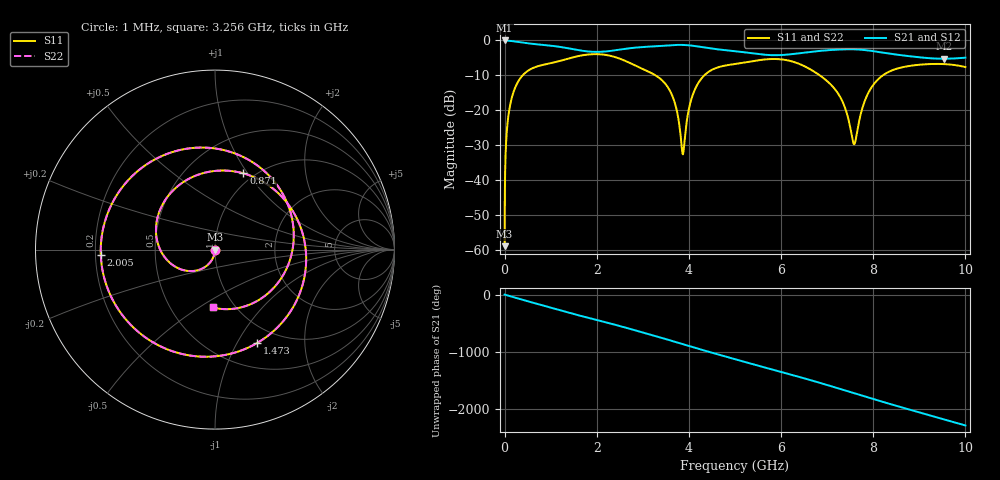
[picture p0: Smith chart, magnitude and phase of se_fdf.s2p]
!Created with skrf (http://scikit-rf.org).
# GHz S RI R 50.0
!freq ReS11 ImS11 ReS21 ImS21 ReS12 ImS12 ReS22 ImS22
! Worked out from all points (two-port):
!   10000 points, 1 MHz to 10 GHz, reference 50 ohm
!   highest |S21| = 0.00 dB at 1 MHz (marker M1); lowest = -5.2 dB at 9.53 GHz (marker M2)
!   |S21| within 3 dB of the highest: start of sweep to 1.716 GHz; 2.294 GHz to 4.951 GHz (2.657 GHz wide, 73.3 % of centre)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
!   lowest |S11| = -58.8 dB at 1 MHz (marker M3), VSWR 1.00, Z = 50 - j0.114 ohm
!   |S11| at or under -10 dB: start of sweep to 391.1 MHz; 3.278 GHz to 4.333 GHz (1.055 GHz wide, 27.7 % of centre); 6.842 GHz to 8.207 GHz (1.366 GHz wide, 18.1 % of centre)
!   |S22| runs from -58.8 to -3.9 dB; largest |S21 - S12| = 1.1e-15
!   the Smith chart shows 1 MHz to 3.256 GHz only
!   S11 on the Smith chart (normalised r, x): 1 MHz: 1.00, -0.00; 871 MHz: 0.89, +0.96; 1.473 GHz: 0.79, -1.22; 2.005 GHz: 0.22, -0.02; 3.256 GHz: 0.79, -0.57
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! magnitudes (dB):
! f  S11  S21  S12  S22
! 1 MHz  -58.8  0.0  0.0  -58.8
! 65 MHz  -23.6  -0.1  -0.1  -23.6
! 176 MHz  -15.5  -0.2  -0.2  -15.5
! 427 MHz  -9.5  -0.7  -0.7  -9.5
! 871 MHz  -6.9  -1.3  -1.3  -6.9
! 1.473 GHz  -4.9  -2.5  -2.5  -4.9
! 1.668 GHz  -4.3  -2.9  -2.9  -4.3
! 2.005 GHz  -3.9  -3.3  -3.3  -3.9
! 3.256 GHz  -9.8  -1.7  -1.7  -9.8
! 3.334 GHz  -10.5  -1.6  -1.6  -10.5
! 3.662 GHz  -16.6  -1.3  -1.3  -16.6
! 3.869 GHz  -32.6  -1.3  -1.3  -32.6
! 4.029 GHz  -18.0  -1.4  -1.4  -18.0
! 4.216 GHz  -11.9  -1.8  -1.8  -11.9
! 5.001 GHz  -6.7  -3.1  -3.1  -6.7
! 6.667 GHz  -8.5  -3.2  -3.2  -8.5
! 7.262 GHz  -15.7  -2.6  -2.6  -15.7
! 7.585 GHz  -29.7  -2.5  -2.5  -29.7
! 7.888 GHz  -15.1  -2.9  -2.9  -15.1
! 8.334 GHz  -9.0  -3.7  -3.7  -9.0
! 9.53 GHz  -6.8  -5.2  -5.2  -6.8
! 10 GHz  -7.6  -4.9  -4.9  -7.6
